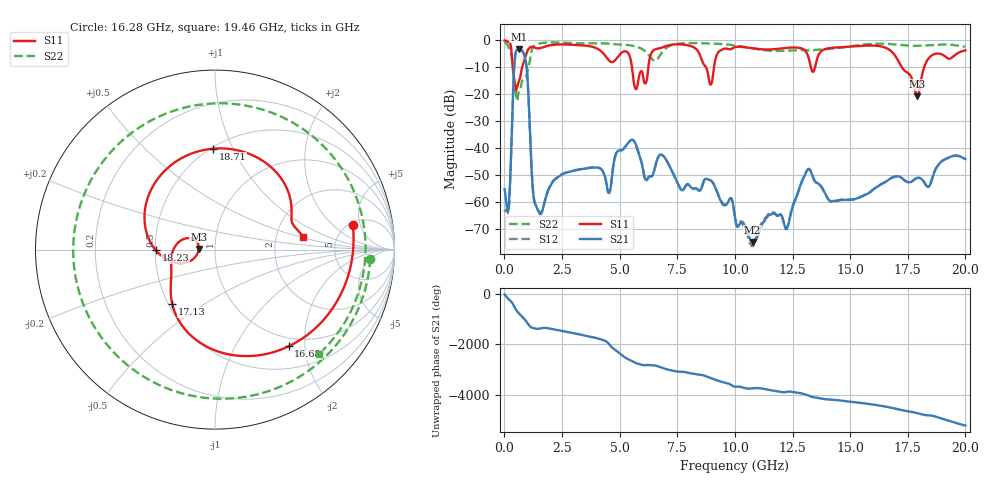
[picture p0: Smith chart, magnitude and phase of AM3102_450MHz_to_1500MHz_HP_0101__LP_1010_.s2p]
!Agilent Technologies,E8364B,MY43040894,A.07.50.67
!Agilent E8364B: A.07.50.67
!Date: Thursday, January 11, 2018 05:42:26
!Correction: S11(Full 2 Port(1,2))
!S21(Full 2 Port(1,2))
!S12(Full 2 Port(1,2))
!S22(Full 2 Port(1,2))
!S2P File: Measurements: S11, S21, S12, S22:
# Hz S  dB  R 50
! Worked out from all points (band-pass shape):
!   1601 points, 10 MHz to 20 GHz, reference 50 ohm
!   highest |S21| = -3.23 dB at 622.2 MHz (marker M1); lowest = -74.9 dB at 10.77 GHz (marker M2)
!   |S21| within 3 dB of the highest: 461.8 MHz to 889.1 MHz (427.3 MHz wide, 63.3 % of centre)
!   lowest |S11| = -20.8 dB at 17.91 GHz (marker M3), VSWR 1.20, Z = 41.7 + j0.283 ohm
!   |S11| at or under -10 dB: 365.5 MHz to 770.4 MHz (404.9 MHz wide, 71.3 % of centre); 5.537 GHz to 6.246 GHz (709.7 MHz wide, 12 % of centre); 17.24 GHz to 18.21 GHz (972.4 MHz wide, 5.49 % of centre)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
!   |S22| runs from -22.5 to -0.7 dB; largest |S21 - S12| = 0.0042
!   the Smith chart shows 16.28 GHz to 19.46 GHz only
!   S11 on the Smith chart (normalised r, x): 16.28 GHz: 5.38, +3.77; 16.68 GHz: 0.85, -1.69; 17.13 GHz: 0.52, -0.37; 18.23 GHz: 0.50, -0.00; 18.71 GHz: 0.51, +0.84; 19.46 GHz: 2.86, +0.54
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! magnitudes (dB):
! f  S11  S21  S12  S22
! 10 MHz  -0.1  -55.3  -62.9  -0.7
! 184.9 MHz  -0.6  -62.3  -63.2  -2.5
! 447.3 MHz  -15.6  -7.5  -7.5  -15.9
! 622.2 MHz  -15.4  -3.2  -3.2  -19.2
! 934.5 MHz  -5.5  -8.1  -8.1  -13.5
! 1.247 GHz  -2.5  -56.5  -56.4  -2.5
! 1.459 GHz  -3.0  -63.2  -63.0  -1.3
! 3.346 GHz  -1.9  -47.9  -47.8  -1.1
! 5.707 GHz  -18.1  -38.8  -38.8  -2.3
! 6.682 GHz  -3.1  -43.2  -43.3  -6.5
! 8.943 GHz  -16.5  -52.1  -52.0  -1.2
! 10.01 GHz  -2.5  -65.8  -65.6  -1.9
! 10.77 GHz  -3.0  -74.9  -76.4  -2.9
! 13.34 GHz  -11.3  -49.8  -49.8  -3.7
! 16.28 GHz  -2.2  -53.9  -53.8  -1.2
! 16.68 GHz  -3.4  -51.7  -51.7  -1.4
! 17.13 GHz  -8.3  -50.6  -50.6  -1.7
! 17.91 GHz  -20.8  -51.1  -51.2  -2.0
! 18.23 GHz  -9.6  -52.9  -53.0  -2.0
! 18.71 GHz  -5.0  -47.7  -47.8  -1.7
! 19.46 GHz  -6.1  -43.0  -43.0  -1.7
! 20 GHz  -3.7  -44.1  -44.0  -2.4
